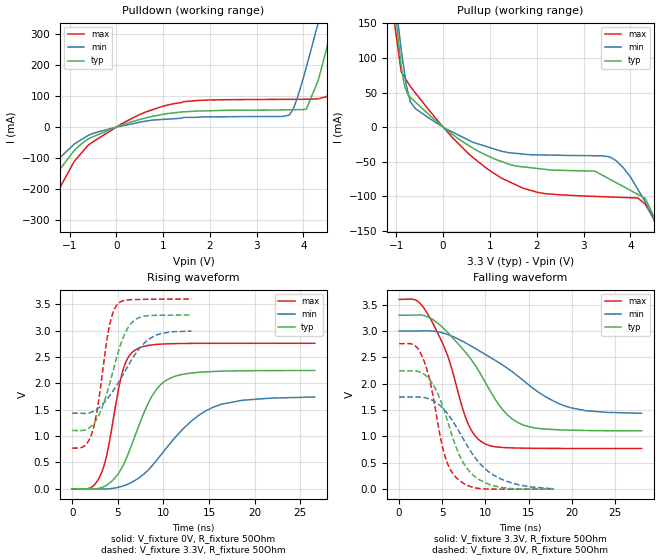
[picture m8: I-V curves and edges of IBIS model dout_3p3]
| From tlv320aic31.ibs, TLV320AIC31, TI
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|   dout_3p3 Model
[Model]   dout_3p3
Model_type   Output
Polarity   Non-Inverting
Vmeas = 1.65
Vref = 1.65
Cref = 10pF
Rref = 50
|   typ   min   max
|   (nom PVT)   (fast PVT)   (slow PVT)
|C_comp from frequency sweep method (F=25MHz)
|C_comp   1.909e-11   1.900e-11   1.955e-11
|ON state : BUFFER OUTPUT TURNED HIGH
|C_comp   1.909e-11   1.900e-11   1.955e-11
|OFF state: BUFFER OUTPUT TURNED LOW
|C_comp   1.628e-11   1.447e-11   1.842e-11
|C_comp from LC tank measurement(L=1nH)
|Resonant Frequency(Hz)   1.920e+09   1.940e+09   1.900e+09
C_comp   6.878e-12   6.737e-12   7.024e-12
|ON state : BUFFER OUTPUT TURNED HIGH
|Resonant Frequency(Hz)   1.920e+09   1.940e+09   1.900e+09
|C_comp   6.878e-12   6.737e-12   7.024e-12
|OFF state: BUFFER OUTPUT TURNED LOW
|Resonant Frequency(Hz)   2.080e+09   2.090e+09   2.070e+09
|C_comp   5.861e-12   5.805e-12   5.917e-12
| Where nom  PVT is Nominal Process, 3.3V, 26C
|   Fast PVT is Strong Process,  3.6V, -40C
|   Slow PVT is Weak Process,   3V, 86C
[Voltage Range]   3.3   3   3.6
|Ambient Temperature   25   85   -40
|Junction Temperature
[Temperature Range]   26   86   -40
[Pullup Reference]   3.3   3   3.6
[Pulldown Reference]   0   0   0
[Power Clamp Reference]   3.3   3   3.6
[GND Clamp Reference]   0   0   0
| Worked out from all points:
|   slope of the pulldown table from 0 to 0.495 V, typ, clamps not added: 20.4 ohm
|   slope of the pullup table from 0 to 0.495 V, typ, clamps not added: 20.2 ohm
|   falling waveform, V_fixture 3.3V, R_fixture 50Ohm: 20-80 % time 5.56ns typ, 8.34ns min, 3.5ns max; typ from 3.3 V to 1.11 V
|   rising waveform, V_fixture 0V, R_fixture 50Ohm: 20-80 % time 3.28ns typ, 5.58ns min, 1.83ns max; typ from 0 V to 2.24 V
|   rising waveform, V_fixture 3.3V, R_fixture 50Ohm: 20-80 % time 2.29ns typ, 3.43ns min, 1.45ns max; typ from 1.1 V to 3.3 V
|   falling waveform, V_fixture 0V, R_fixture 50Ohm: 20-80 % time 3.11ns typ, 4.44ns min, 2.13ns max; typ from 2.25 V to 0.001 V
[Pulldown]
|   Voltage   I(typ)   I(min)   I(max)
-3.3V     -1.438A    -1.188A    -1.781A
-1.994V   -464.2mA   -346.6mA   -625.7mA
-1.656V   -253.8mA   -174.2mA   -369.2mA
-465mV    -28.97mA   -18.63mA   -44.06mA
1.246V    46.31mA    27.19mA    76.19mA
3.684V    55.88mA    38.18mA    89.54mA
4.062V    58.36mA    194.3mA    89.91mA
4.314V    150.4mA    336.2mA    91.28mA
4.507V    260.5mA    449.4mA    100.3mA
4.694V    377.7mA    562.3mA    191.8mA
5.166V    672.8mA    846.6mA    504.7mA
6.6V      1.613A     1.739A     1.547A
[Pullup]
|   Voltage   I(typ)   I(min)   I(max)
-3.3V     1.671A     1.612A     1.822A
-1.04V    176.8mA    195.6mA    150.7mA
-896.4mV  87.61mA    111.3mA    79.9mA
-821.7mV  58.54mA    76.66mA    71.79mA
-702mV    42.98mA    36.58mA    58.79mA
-591mV    36.08mA    26.62mA    49.28mA
633.6mV   -30.34mA   -21.85mA   -43.8mA
1.706V    -57.47mA   -38.93mA   -88.32mA
3.591V    -76.44mA   -44.11mA   -101.1mA
4.162V    -97.38mA   -90.12mA   -102.8mA
4.713V    -169.8mA   -178.4mA   -177.1mA
6.6V      -1.372A    -1.338A    -1.416A
[Ramp]
R_load = 50
|   typ   min   max
dV/dt_r   1.3468/3.27193e-09   1.04865/5.61481e-09   1.65639/1.82217e-09
dV/dt_f   1.31652/5.55613e-09   0.939151/8.37139e-09   1.69697/3.4918e-09
[Falling Waveform]
V_fixture = 3.3V
V_fixture_min = 3V
V_fixture_max = 3.6V
R_fixture = 50Ohm
|   Time   V(typ)   V(min)   V(max)
0s        3.3V       3V         3.6V
1.96ns    3.305V     3V         3.587V
3.345ns   3.268V     3.005V     3.315V
5.565ns   2.982V     2.939V     2.557V
7.98ns    2.54V      2.749V     1.246V
9.91ns    2.048V     2.565V     862.7mV
12.03ns   1.502V     2.351V     790.8mV
14.41ns   1.217V     2.059V     778.2mV
19.88ns   1.119V     1.545V     772.6mV
28.11ns   1.107V     1.441V     771.8mV
[Rising Waveform]
V_fixture = 0V
V_fixture_min = 0V
V_fixture_max = 0V
R_fixture = 50Ohm
|   Time   V(typ)   V(min)   V(max)
0s        1.237nV    4.434nV    833.1pV
1.965ns   -6.487mV   -1.987mV   14.13mV
3.07ns    14.16mV    -5.47mV    249.7mV
3.82ns    73.98mV    -2.443mV   670mV
5.56ns    437.7mV    52.53mV    2.253V
7.24ns    1.172V     198mV      2.667V
9.22ns    1.885V     534.2mV    2.738V
11.31ns   2.137V     979.9mV    2.754V
16.42ns   2.231V     1.606V     2.76V
26.58ns   2.244V     1.74V      2.761V
[Rising Waveform]
V_fixture = 3.3V
V_fixture_min = 3V
V_fixture_max = 3.6V
R_fixture = 50Ohm
|   Time   V(typ)   V(min)   V(max)
0s        1.105V     1.433V     771.7mV
1.33ns    1.111V     1.43V      812.8mV
2.175ns   1.203V     1.458V     1.064V
2.76ns    1.346V     1.517V     1.531V
4.11ns    1.999V     1.767V     3.121V
4.95ns    2.543V     1.984V     3.499V
6.055ns   3.041V     2.313V     3.583V
7.04ns    3.224V     2.589V     3.59V
9.215ns   3.291V     2.916V     3.597V
13.08ns   3.297V     2.992V     3.599V
[Falling Waveform]
V_fixture = 0V
V_fixture_min = 0V
V_fixture_max = 0V
R_fixture = 50Ohm
|   Time   V(typ)   V(min)   V(max)
0s        2.245V     1.749V     2.761V
1.65ns    2.245V     1.749V     2.745V
2.61ns    2.208V     1.745V     2.538V
3.6ns     2.064V     1.705V     2.031V
5.2ns     1.502V     1.513V     688.2mV
5.91ns    1.133V     1.365V     379.2mV
6.64ns    779.3mV    1.179V     215.5mV
8.33ns    303.6mV    709.4mV    46.73mV
11.01ns   63.59mV    260.2mV    1.011mV
17.95ns   582.5uV    6.607mV    95.01uV
